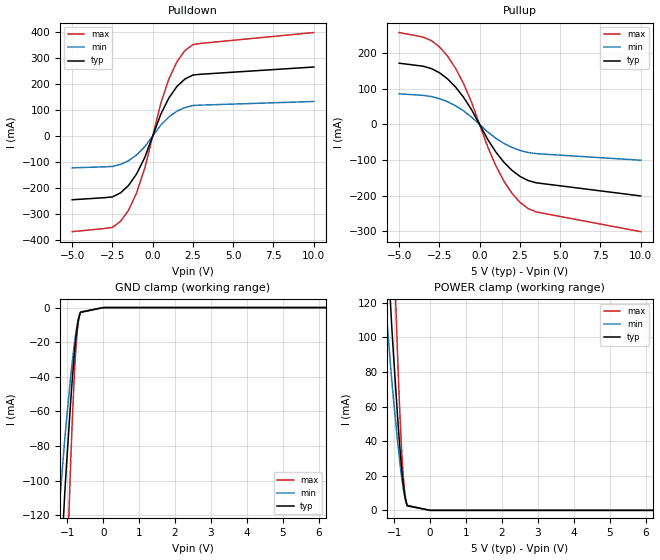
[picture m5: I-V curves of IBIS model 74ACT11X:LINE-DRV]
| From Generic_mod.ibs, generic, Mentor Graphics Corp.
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[Model]   74ACT11X:LINE-DRV
Model_type   I/O
Polarity   Non-Inverting
Vinl  =   0.800V
Vinh  =   2.000V
Vmeas =   1.500V
Cref  =  50.000pF
Rref  =   1.000kOhm
Vref  =   0.000V
|   typ   min   max
C_comp   10.000pF   5.000pF   15.000pF
[Voltage Range]   5.000V   4.500V   5.500V
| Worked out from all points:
|   slope of the pulldown table from 0 to 0.75 V, typ, clamps not added: 6.55 ohm
|   slope of the pullup table from 0 to 0.75 V, typ, clamps not added: 12.7 ohm
[Pulldown]
| Voltage   I(typ)   I(min)   I(max)
-5V       -245.3mA   -122.6mA   -367.9mA
-2.5V     -234.3mA   -117.2mA   -351.5mA
-2V       -218.9mA   -109.4mA   -328.3mA
-1.5V     -190.1mA   -95.06mA   -285.2mA
-1V       -145.8mA   -72.88mA   -218.6mA
-500mV    -83.33mA   -41.67mA   -125mA
500mV     83.33mA    41.67mA    125mA
1V        145.8mA    72.88mA    218.6mA
1.5V      190.1mA    95.06mA    285.2mA
2V        218.9mA    109.4mA    328.3mA
3V        237.4mA    118.7mA    356.1mA
10V       265.1mA    132.6mA    397.7mA
[Pullup]
| Voltage   I(typ)   I(min)   I(max)
-5V       172.2mA    86.12mA    258.4mA
-3V       157.2mA    78.61mA    235.8mA
-2V       128.4mA    64.22mA    192.7mA
-1.5V     105.6mA    52.79mA    158.4mA
-1V       76.76mA    38.38mA    115.1mA
-500mV    41.67mA    20.83mA    62.5mA
500mV     -41.67mA   -20.83mA   -62.5mA
1V        -76.76mA   -38.38mA   -115.1mA
1.5V      -105.6mA   -52.79mA   -158.4mA
2.5V      -145.6mA   -72.78mA   -218.3mA
3.5V      -163.6mA   -81.82mA   -245.5mA
10V       -200.7mA   -100.3mA   -301mA
[GND Clamp]
| Voltage   I(typ)   I(min)   I(max)
-5V       -1.627A    -1.09A     -3.228A
-1.069V   -106.5mA   -75.37mA   -190.7mA
-1.017V   -89.04mA   -63.62mA   -156.6mA
-907.7mV  -54.62mA   -40.28mA   -90.16mA
-855.5mV  -39.76mA   -30.06mA   -62.37mA
-808.2mV  -27.74mA   -21.64mA   -40.79mA
-768.6mV  -19.05mA   -15.4mA    -26.1mA
-749.3mV  -15.39mA   -12.7mA    -20.27mA
-692.5mV  -7.18mA    -6.349mA   -8.397mA
-634.6mV  -2.693mA   -2.54mA    -2.876mA
0V        0A         0A         0A
10V       0A         0A         0A
[POWER Clamp]
| Voltage   I(typ)   I(min)   I(max)
-5V       1.627A     1.09A      3.228A
-1.069V   106.5mA    75.37mA    190.7mA
-1.017V   89.04mA    63.62mA    156.6mA
-907.7mV  54.62mA    40.28mA    90.16mA
-855.5mV  39.76mA    30.06mA    62.37mA
-808.2mV  27.74mA    21.64mA    40.79mA
-768.6mV  19.05mA    15.4mA     26.1mA
-749.3mV  15.39mA    12.7mA     20.27mA
-692.5mV  7.18mA     6.349mA    8.397mA
-634.6mV  2.693mA    2.54mA     2.876mA
0V        0A         0A         0A
10V       0A         0A         0A
[Ramp]
|   typ   min   max
dV/dt_r   2.375V/1.440ns   1.699V/2.592ns   2.820V/1.056ns
dV/dt_f   2.672V/1.140ns   2.121V/2.052ns   3.056V/836.000ps
R_load =  50.000Ohm
|------------------- End of 74ACT11X:LINE-DRV ---------------------------------
